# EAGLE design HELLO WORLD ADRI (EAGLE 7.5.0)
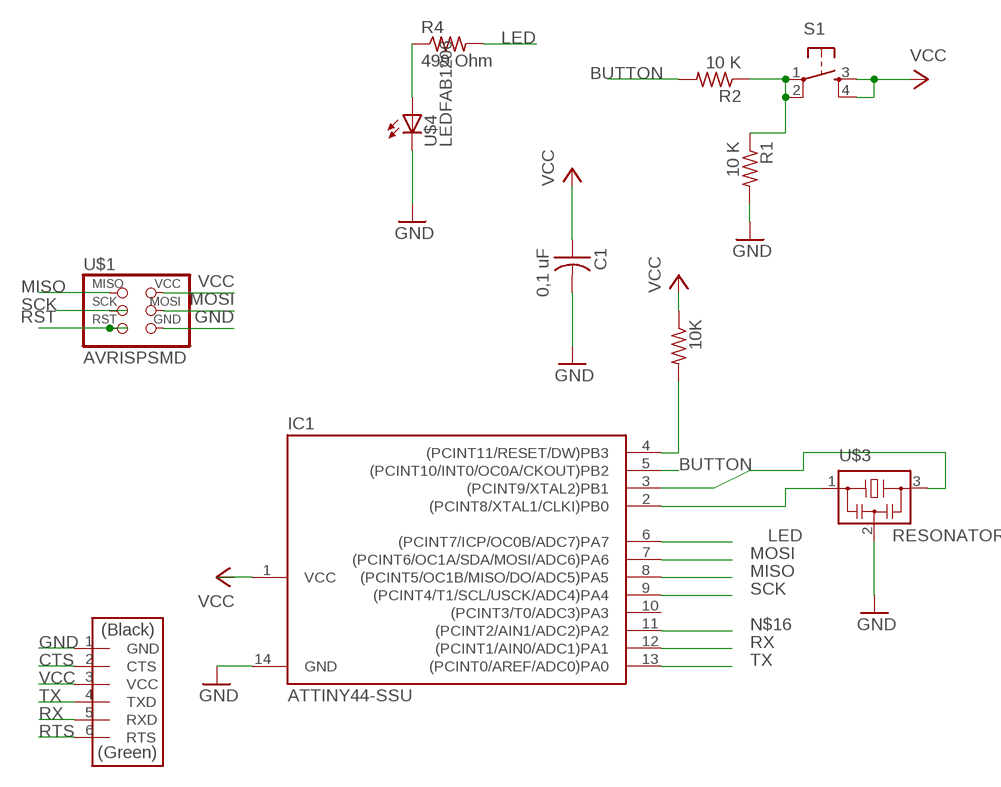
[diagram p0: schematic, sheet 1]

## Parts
10K  RES-US1206  [R1206]
C1  0,1 uF  CAP-US1206FAB  [C1206FAB]
IC1  ATTINY44-SSU  [SOIC14]
R1  10 K  RES-US1206  [R1206]
R2  10 K  RES-US1206  [R1206]
R4  499 Ohm  RES-US1206  [R1206]
S1  6MM_SWITCH6MM_SWITCH  [6MM_SWITCH]
U$1  AVRISPSMD  [2X03SMD]
U$2  FTDI-SMD-HEADER  [1X06SMD]
U$3  RESONATOR  [EFOBM]
U$4  LEDFAB1206  [LED1206FAB]

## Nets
BUTTON: IC1.5((PCINT10/INT0/OC0A/CKOUT)PB2) R2.2
CTS: U$2.2(CTS)
GND: C1.2 IC1.14(GND) R1.2 U$1.6(GND) U$2.1(GND) U$3.2 U$4.2(C)
LED: IC1.6((PCINT7/ICP/OC0B/ADC7)PA7) R4.2
MISO: IC1.8((PCINT5/OC1B/MISO/DO/ADC5)PA5) U$1.1(MISO)
MOSI: IC1.7((PCINT6/OC1A/SDA/MOSI/ADC6)PA6) U$1.4(MOSI)
N$1: IC1.2((PCINT8/XTAL1/CLKI)PB0) U$3.1
N$2: R4.1 U$4.1(A)
N$3: 10K.2 IC1.4((PCINT11/RESET/DW)PB3)
N$4: R1.1 R2.1 S1.1(P) S1.2(P1)
N$10: IC1.3((PCINT9/XTAL2)PB1) U$3.3
N$16: IC1.11((PCINT2/AIN1/ADC2)PA2)
RST: U$1.5(RST)
RTS: U$2.6(RTS)
RX: IC1.12((PCINT1/AIN0/ADC1)PA1) U$2.5(RXD)
SCK: IC1.9((PCINT4/T1/SCL/USCK/ADC4)PA4)
TX: IC1.13((PCINT0/AREF/ADC0)PA0) U$2.4(TXD)
VCC: 10K.1 C1.1 IC1.1(VCC) S1.3(S) S1.4(S1) U$1.2(VCC) U$2.3(VCC)
Unconnected: IC1.10((PCINT3/T0/ADC3)PA3) U$1.3(SCK)

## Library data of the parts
10K R1 R2 R4 = fab:RES-US: Resistor (US Symbol)
C1 = fab:CAP-US
IC1 = fab:ATTINY44
S1 = fab:6MM_SWITCH: OMRON SWITCH
U$1 = fab:AVRISP
U$2 = fab:FTDI-SMD-HEADER
U$3 = fab:RESONATOR
U$4 = fab:LED: LED

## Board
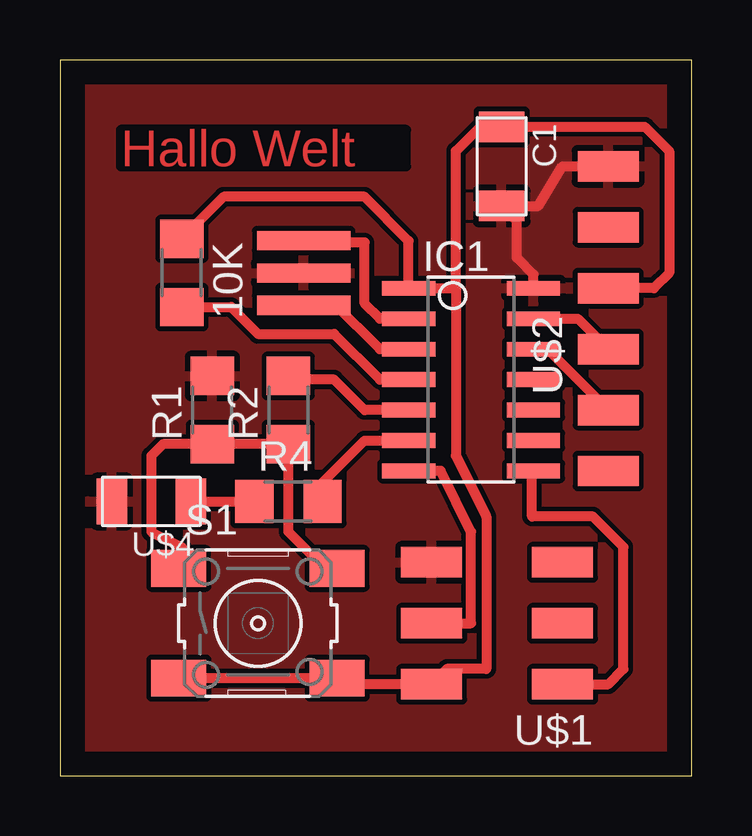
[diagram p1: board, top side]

Size 26.34 x 29.84 mm. Coordinates in mm from the lower left corner, seen from the top.
Outline: 0,0 26.34,0 26.34,29.84 0,29.84 0,0
Copper layers (1*16): Top 0.035mm / dielectric 1.5mm / Bottom 0.035mm
Design rules "default": minimum track width 10mil, minimum drill 24mil, track to track 8mil, track to pad 8mil, pad to pad 8mil, via to via 8mil, smd to smd 8mil, copper to edge 40mil, drill to drill 8mil, minimum pad ring 10mil, minimum via ring 8mil, stop-mask expansion 4mil, vias tented up to drill 0mil, thermal gap 10mil

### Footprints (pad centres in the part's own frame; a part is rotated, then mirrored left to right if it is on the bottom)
R1206 = smd 1.6 x 1.803: 1 -1.422,0; 2 1.422,0
C1206FAB = smd 1.27 x 1.905: 1 -1.651,0; 2 1.651,0
SOIC14 = smd 0.61 x 2.21: 1 -3.81,-2.603; 2 -2.54,-2.603; 3 -1.27,-2.603; 4 0,-2.603; 5 1.27,-2.603; 6 2.54,-2.603; 7 3.81,-2.603; 8 3.81,2.603; 9 2.54,2.603; 10 1.27,2.603; 11 0,2.603; 12 -1.27,2.603; 13 -2.54,2.603; 14 -3.81,2.603
6MM_SWITCH = smd 2.286 x 1.524: 1 -3.302,2.286; 2 3.302,2.286; 3 -3.302,-2.286; 4 3.302,-2.286
2X03SMD = smd 2.54 x 1.27: 1 -2.54,2.54; 2 2.92,2.54; 3 -2.54,0; 4 2.92,0; 5 -2.54,-2.54; 6 2.92,-2.54
1X06SMD = smd 2.54 x 1.27: 1 0,6.35; 2 0,3.81; 3 0,1.27; 4 0,-1.27; 5 0,-3.81; 6 0,-6.35
EFOBM = smd 0.8 x 3.9: 1 -1.35,0; 2 0,0; 3 1.35,0
LED1206FAB = smd 1.27 x 1.905: 1 -1.651,0; 2 1.651,0

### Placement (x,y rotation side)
10K  5.08,20.96 270 top
C1  18.41,25.4 270 top
IC1  17.15,16.51 270 top
R1  6.35,15.24 90 top
R2  9.53,15.24 90 top
R4  9.53,11.43 0 top
S1  8.26,6.35 0 top
U$1  18.41,6.35 180 top
U$2  22.86,19.05 0 top
U$3  10.16,20.96 270 top
U$4  3.81,11.43 180 top

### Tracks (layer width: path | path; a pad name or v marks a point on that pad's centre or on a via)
BUTTON
  Top 0.406: IC1.5 12.7,15.24 11.43,16.51 9.68,16.51 R2.2
GND
  Top 0.406: IC1.14 19.75,20.89 19.05,21.59 19.05,23.11 C1.2 19.94,23.75 20.95,25.4 U$2.1
  pour Top: 0.63,29.21 0.63,0 26.67,0 26.67,29.21
LED
  Top 0.406: R4.2 10.95,12.22 12.7,13.97 IC1.6
MISO
  Top 0.406: U$1.1 22.86,3.81 23.5,4.45 23.5,9.53 22.23,10.79 19.69,10.79 19.69,12.64 IC1.8
MOSI
  Top 0.406: U$1.4 17.15,6.35 17.15,10.16 15.87,12.7 IC1.7
N$1
  Top 0.406: IC1.2 13.33,19.05 12.7,19.69 12.7,22.23 10.08,22.23 | 9.53,22.23 10.08,22.23 | 10.08,22.23 U$3.1
N$2
  Top 0.406: U$4.1 R4.1
N$3
  Top 0.406: IC1.4 13.33,16.51 11.43,18.42 8.26,18.42 7.14,19.53 10K.2
N$4
  Top 0.406: 4.95,9.02 S1.1 5.08,8.76 5.08,9.53 3.81,10.16 3.81,13.33 4.29,13.82 R1.1 R2.1 9.53,10.16 11.05,8.64 S1.2
N$10
  Top 0.406: IC1.3 13.33,17.78 11.43,19.69 10.79,19.69 | U$3.3 10.71,19.61 10.79,19.69 | 10.79,19.69 9.53,19.69
RX
  Top 0.406: IC1.12 20.32,17.78 U$2.5
TX
  Top 0.406: IC1.13 21.59,19.05 U$2.4
VCC
  Top 0.406: 10K.1 6.83,24.13 12.7,24.13 14.54,22.29 IC1.1 16.51,20.32 | 22.23,20.32 U$2.3 24.77,20.32 25.4,20.96 25.4,26.04 24.38,27.05 C1.1 18.16,27.3 17.78,27.3 16.51,26.04 16.51,20.32 | 16.51,20.32 16.51,13.33 17.78,10.79 17.78,4.45 16.13,4.45 U$1.2 11.81,3.81 S1.4 S1.3

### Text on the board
Top: Hallo Welt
